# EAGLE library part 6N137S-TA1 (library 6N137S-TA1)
High Speed Optocouplers High Speed 10MBd LogicGate Output Source: Datasheet
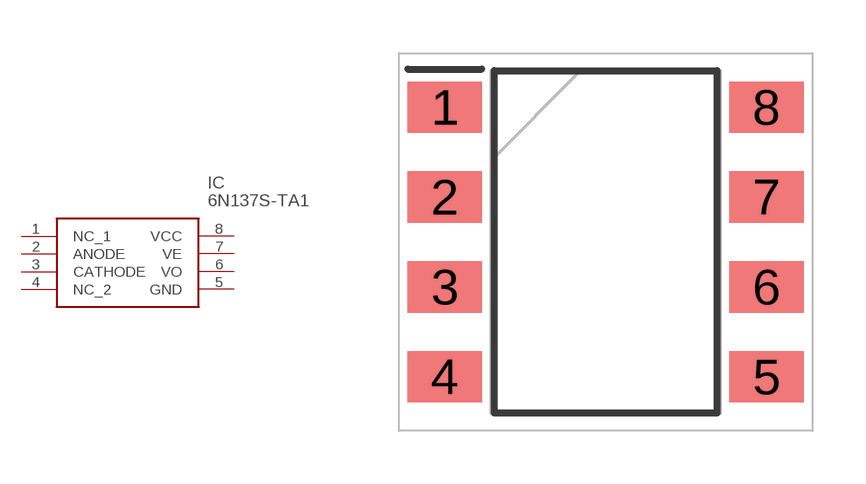
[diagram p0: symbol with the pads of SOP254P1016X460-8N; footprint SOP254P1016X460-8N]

Designator prefix IC

## 6N137S-TA1 (Description: High Speed Optocouplers High Speed 10MBd LogicGate Output; Height: 4.6mm; Manufacturer_Name: Lite-On; Manufacturer_Part_Number: 6N137S-TA1; Mouser_Part_Number: 859-6N137STA1; Mouser_Price-Stock: https://www.mouser.co.uk/ProductDetail/Lite-On/6N137S-TA1?qs=PByDJ0nQNwrChwHSrgNi1w%3D%3D)  [SOP254P1016X460-8N]
1  NC_1
2  ANODE
3  CATHODE
4  NC_2
5  GND
6  VO
7  VE
8  VCC

## Footprint SOP254P1016X460-8N (pad centres in mm)
6N137S-TA1
smd 2.1 x 1.45: 1 -4.55,3.81; 2 -4.55,1.27; 3 -4.55,-1.27; 4 -4.55,-3.81; 5 4.55,-3.81; 6 4.55,-1.27; 7 4.55,1.27; 8 4.55,3.81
